FUNCTION_BLOCK MIS_ProfileHoming
VAR_INPUT
	eCmd : eCommand;
	iHomingMode : INT;			//CANopen homing mode
	rVelocityRpmSearch : REAL; 	//Search velocity 
	rVelocityRpmCrawl : REAL; 	//Crawl velocity
	rAccellRpms : REAL; 		//Homing Acceleration 	
	rHomingtorquePct : REAL; 	//Homing torque in percent of set max 	
	lrHomePos : LREAL;			//Homing pos 
	
END_VAR
VAR_IN_OUT
	stMisMotorLocal : stMisMotor;	
END_VAR
VAR_OUTPUT
	eError : eErrorCodesMIS;
	eStat: ESTATUS;
END_VAR	
VAR
	
	//Io 
	bHomingCompleteSuccess : BOOL;
	bHomingCompleteFailed : BOOL;
	bHomingStart : BOOL;
	
	//Variables	
	iState : INT;
	SDO_WRITE : SDOwrite;
	WriteError: DWORD;
 	WriteData:ARRAY[0..255] OF BYTE;
END_VAR

IF eCmd = eCommand.Reset THEN
	eError := eErrorCodesMIS.None;
	iState := 0;
	eStat := eStatus.Done;
	RETURN;
END_IF;

bHomingCompleteSuccess := ((stMisMotorLocal.uiStatus AND 16#1000) > 0);
bHomingCompleteFailed := ((stMisMotorLocal.uiStatus AND 16#2000) > 0);


CASE iState OF 
0:
	CASE eCmd OF
	eCommand.Run:
		eStat := eStatus.Running;
		eError := eErrorCodesMIS.None;
		iState := 100;
	END_CASE

100://Write Homing mode 
	DwordToByteArray(diValue := iHomingMode,Datalenght := 1,DataOut := WriteData);
	SDO_WRITE(StartWriting := TRUE,CO_Index := 16#6098, CO_SubIndex := 0, DataLength := DwordToByteArray.Datalenght,
	PortNr := 16#1000 + stMisMotorLocal.wNodeId, WriteData := WriteData, ADSNetID:= stMisMotorLocal.ADSNetID);
	IF SDO_WRITE.WriteDataFinished THEN
		SDO_WRITE(StartWriting := FALSE);
		WriteError := SDO_WRITE.Error;
		IF WriteError <> 0 THEN 
			eError := eErrorCodesMIS.ModeHomeErrWritingmode;
			iState := 1000; 
		ELSE
			iState := 110;
		END_IF;
	END_IF


110: //Homing velocity
	DwordToByteArray(diValue := ANY_TO_DINT(rVelocityRpmSearch * ANY_TO_REAL(stMisMotorLocal.diRpmConversion)),Datalenght := 4,DataOut := WriteData);
	SDO_WRITE(StartWriting := TRUE,CO_Index := 16#6099, CO_SubIndex := 1, DataLength := DwordToByteArray.Datalenght,
	PortNr := 16#1000 + stMisMotorLocal.wNodeId, WriteData := WriteData, ADSNetID:= stMisMotorLocal.ADSNetID);
	IF SDO_WRITE.WriteDataFinished THEN
		SDO_WRITE(StartWriting := FALSE);
		WriteError := SDO_WRITE.Error;
		IF WriteError <> 0 THEN 
			eError := eErrorCodesMIS.ModeHomeErrWritingSpeed;
			iState := 1000; 
		ELSE
			iState := 120;
		END_IF;
	END_IF

	
120://Homing crawl
	DwordToByteArray(diValue := ANY_TO_DINT(rVelocityRpmCrawl * ANY_TO_REAL(stMisMotorLocal.diRpmConversion)),Datalenght := 4,DataOut := WriteData);
	SDO_WRITE(StartWriting := TRUE,CO_Index := 16#6099, CO_SubIndex := 2, DataLength := DwordToByteArray.Datalenght,
	PortNr := 16#1000 + stMisMotorLocal.wNodeId, WriteData := WriteData, ADSNetID:= stMisMotorLocal.ADSNetID);
	IF SDO_WRITE.WriteDataFinished THEN
		SDO_WRITE(StartWriting := FALSE);
		WriteError := SDO_WRITE.Error;
		IF WriteError <> 0 THEN 
			eError := eErrorCodesMIS.ModeHomeErrWritingCrawl;
			iState := 1000; 
		ELSE
			iState := 130;
		END_IF;
	END_IF

130://Homing accel
	DwordToByteArray(diValue := ANY_TO_DINT(rAccellRpms),Datalenght := 4,DataOut := WriteData);
	SDO_WRITE(StartWriting := TRUE,CO_Index := 16#609A, CO_SubIndex := 0, DataLength := DwordToByteArray.Datalenght,
	PortNr := 16#1000 + stMisMotorLocal.wNodeId, WriteData := WriteData, ADSNetID:= stMisMotorLocal.ADSNetID);
	IF SDO_WRITE.WriteDataFinished THEN
		SDO_WRITE(StartWriting := FALSE);
		WriteError := SDO_WRITE.Error;
		IF WriteError <> 0 THEN 
			eError := eErrorCodesMIS.ModeHomeErrWritingAccel;
			iState := 1000; 
		ELSE
			iState := 140;
		END_IF;
	END_IF


140: //Write homing position offset 
	DwordToByteArray(diValue := ANY_TO_DINT(lrHomePos * stMisMotorLocal.lrUnitConversion),Datalenght := 4,DataOut := WriteData);
	SDO_WRITE(StartWriting := TRUE,CO_Index := 16#607C, CO_SubIndex := 0, DataLength := DwordToByteArray.Datalenght,
	PortNr := 16#1000 + stMisMotorLocal.wNodeId, WriteData := WriteData, ADSNetID:= stMisMotorLocal.ADSNetID);
	IF SDO_WRITE.WriteDataFinished THEN
		SDO_WRITE(StartWriting := FALSE);
		WriteError := SDO_WRITE.Error;
		IF WriteError <> 0 THEN 
			eError := eErrorCodesMIS.ModeHomeErrWritingPosOffs;
			iState := 1000; 
		ELSE
			iState := 200;
		END_IF;
	END_IF
	
150://Write homing torque 
	IF 	iHomingMode < 0 THEN
		DwordToByteArray(diValue := ANY_TO_DINT(2047 / 100 * rHomingtorquePct  ),Datalenght := 4,DataOut := WriteData);
		SDO_WRITE(StartWriting := TRUE,CO_Index := 16#607C, CO_SubIndex := 0, DataLength := DwordToByteArray.Datalenght,
		PortNr := 16#1000 + stMisMotorLocal.wNodeId, WriteData := WriteData, ADSNetID:= stMisMotorLocal.ADSNetID);
		IF SDO_WRITE.WriteDataFinished THEN
			SDO_WRITE(StartWriting := FALSE);
			WriteError := SDO_WRITE.Error;
			IF WriteError <> 0 THEN 
				eError := eErrorCodesMIS.ModeHomeErrWritingTorque;
				iState := 1000; 
			ELSE
				iState := 200;
			END_IF;
		END_IF	
	ELSE
		iState := 200; //Skip torque settings when using switch		
	END_IF;
	
200: //Start homing
	bHomingStart := TRUE; //Start homing  sequnce
	iState := iState + 1;

201: //Wait for homing to complete	
	IF bHomingCompleteSuccess THEN
		bHomingStart := FALSE;
		istate := 220;
	ELSIF bHomingCompleteFailed  THEN 
		eError := eErrorCodesMIS.ModeHomeHomingFailed;
		iState := 1000; //Homing Error
	ELSIF eCmd = eCommand.Stop THEN
		bHomingStart := FALSE; //Terminated  by operator
 		stMisMotorLocal.bEnableMotor := FALSE;
		iState := 220;
	END_IF

220: //Done
	eStat := eStatus.Done;	
	IF eCmd <> eCommand.Run THEN 
		iState := 0;		
	END_IF

	
1000: //Error 
	eStat := eStatus.Error;	
	IF eCmd <> eCommand.Run THEN 
		iState := 0;		
	END_IF
END_CASE;



stMisMotorLocal.uiCtrWord := ANY_TO_UINT(CSETBIT32(inVal32 := stMisMotorLocal.uiCtrWord,bitNo := 4,bitVal := bHomingStart));

END_FUNCTION_BLOCK
